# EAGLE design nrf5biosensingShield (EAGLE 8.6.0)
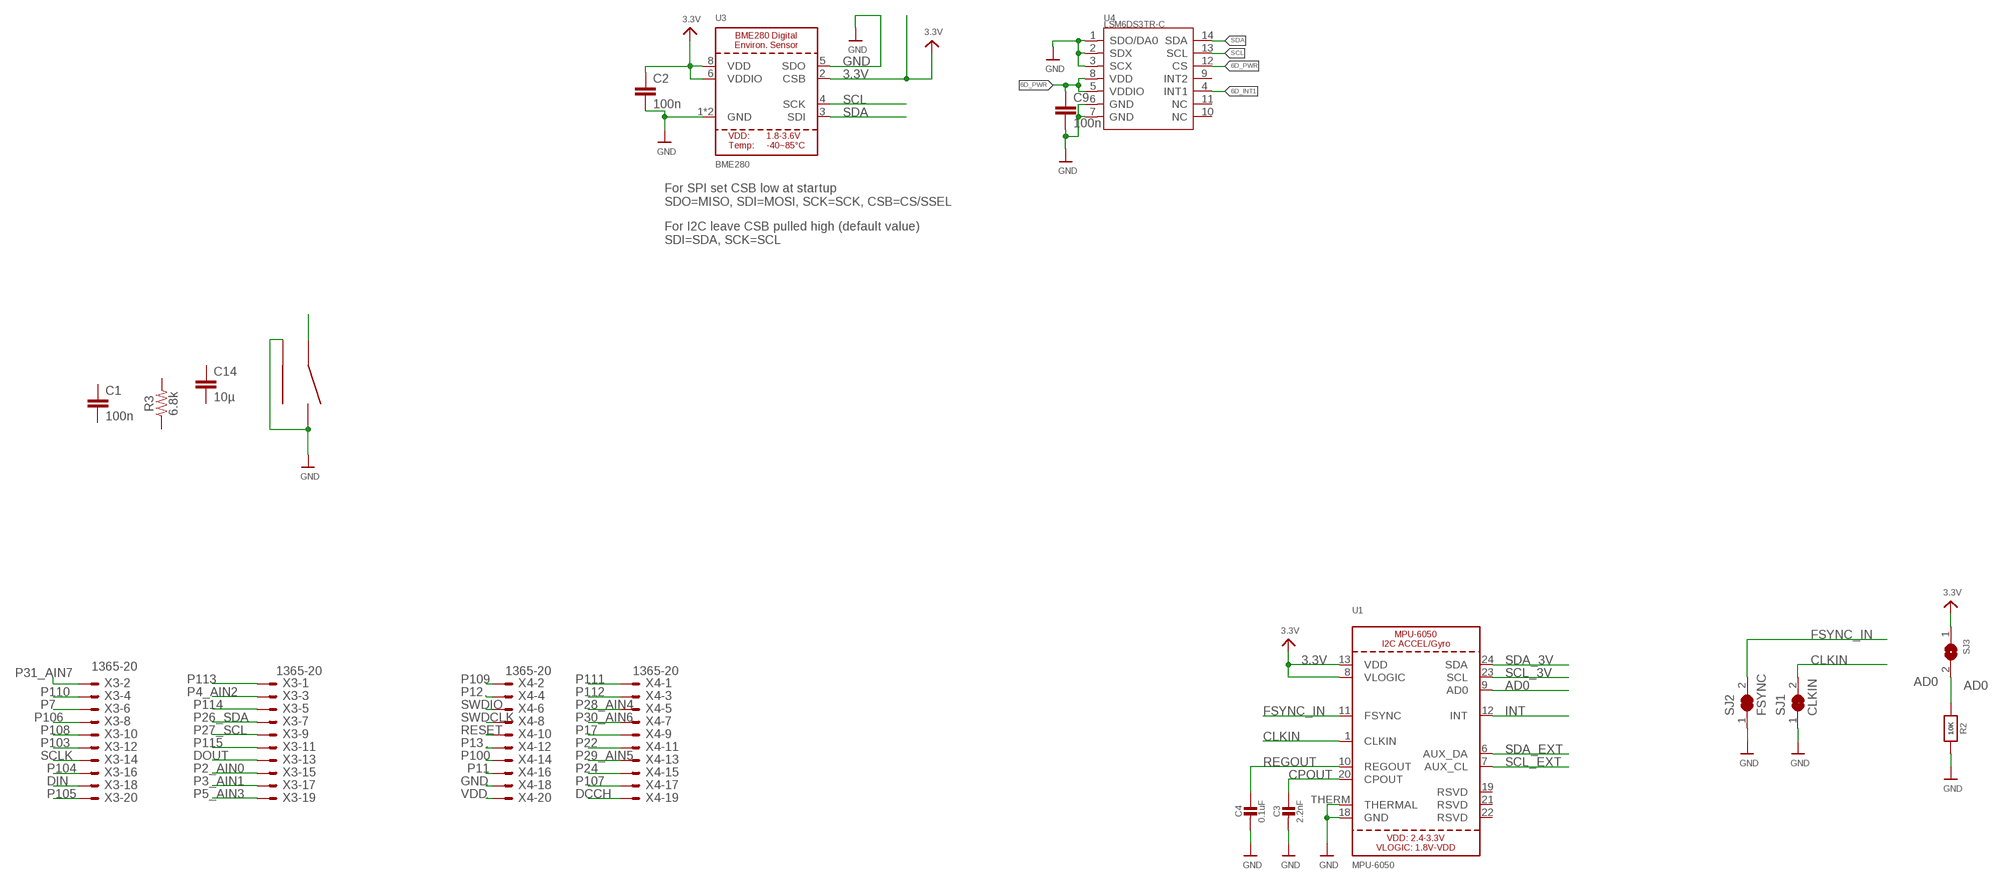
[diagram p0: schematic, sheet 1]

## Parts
C1  100n  CAP-0402-TIGHT  [0402-TIGHT]
C2  100n  C-EUC0402  [C0402]
C3  2.2nF  CAP_CERAMIC0603_NO  [0603-NO]
C4  0.1uF  CAP_CERAMIC0603_NO  [0603-NO]
C9  100n  C-EUC0402  [C0402]
C14  10µ  C-EUC0603  [C0603]
R2  10K  RESISTOR_0603_NOOUT  [0603-NO]
R3  6.8k  RESISTOR0402T  [0402-TIGHT]
S1  LS12T2  [LS12T2]
SJ1  CLKIN  SOLDERJUMPER_CLOSED  [SOLDERJUMPER_CLOSEDWIRE]
SJ2  FSYNC  SOLDERJUMPER_CLOSED  [SOLDERJUMPER_CLOSEDWIRE]
SJ3  SOLDERJUMPER  [SOLDERJUMPER_ARROW_NOPASTE]
U1  MPU-6050  [QFN24_4MM_SMSC]
U3  BME280  [BME280]
U4  LSM6DS3TR-C  SENSOR-LSM6DS3TR-C  [LGA14-0.5-2.5X3X0.86MM]
X3  1365-20  [1365-20]
X4  1365-20  [1365-20]

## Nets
3.3V [power]: C2.1 SJ3.1 U1.8(VLOGIC) U1.13(VDD) U3.2(CSB) U3.6(VDDIO) U3.8(VDD)
6D_INT1: U4.4(INT1)
6D_PWR: C9.1 U4.5(VDDIO) U4.8(VDD) U4.12(CS)
AD0: R2.1 SJ3.2 U1.9(AD0)
BUT: S1.2
CLKIN: SJ1.2 U1.1(CLKIN)
CPOUT: C3.1 U1.20(CPOUT)
DCCH: X4.19
DIN: X3.18
DOUT: X3.13
FSYNC_IN: SJ2.2 U1.11(FSYNC)
GND: C2.2 C3.2 C4.2 C9.2 R2.2 S1.1 S1.FRAME(FRM) SJ1.1 SJ2.1 U1.18(GND) U1.THERM(THERMAL) U3.1(GND) U3.5(SDO) U3.7(GND) U4.1(SDO/DA0) U4.2(SDX) U4.3(SCX) U4.6(GND) U4.7(GND) X4.18
INT: U1.12(INT)
P2_AIN0: X3.15
P3_AIN1: X3.17
P4_AIN2: X3.3
P5_AIN3: X3.19
P7: X3.6
P11: X4.16
P12: X4.4
P13: X4.12
P17: X4.9
P22: X4.11
P24: X4.15
P26_SDA: X3.7
P27_SCL: X3.9
P28_AIN4: X4.5
P29_AIN5: X4.13
P30_AIN6: X4.7
P31_AIN7: X3.2
P100: X4.14
P103: X3.12
P104: X3.16
P105: X3.20
P106: X3.8
P107: X4.17
P108: X3.10
P109: X4.2
P110: X3.4
P111: X4.1
P112: X4.3
P113: X3.1
P114: X3.5
P115: X3.11
REGOUT: C4.1 U1.10(REGOUT)
RESET: X4.10
SCL: U3.4(SCK) U4.13(SCL)
SCL_3V: U1.23(SCL)
SCL_EXT: U1.7(AUX_CL)
SCLK: X3.14
SDA: U3.3(SDI) U4.14(SDA)
SDA_3V: U1.24(SDA)
SDA_EXT: U1.6(AUX_DA)
SWDCLK: X4.8
SWDIO: X4.6
VDD: X4.20
Unconnected: C1.1 C1.2 C14.1 C14.2 R3.1 R3.2 U1.19(RSVD) U1.21(RSVD) U1.22(RSVD) U4.9(INT2) U4.10(NC) U4.11(NC)

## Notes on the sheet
- For SPI set CSB low at startup
  SDO=MISO, SDI=MOSI, SCK=SCK, CSB=CS/SSEL
- For I2C leave CSB pulled high (default value)
  SDI=SDA, SCK=SCL

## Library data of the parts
C1 = SparkFun-Capacitors:CAP
C2 C9 C14 = rcl:C-EU: CAPACITOR, European symbol
C3 C4 = microbuilder:CAP_CERAMIC: Ceramic Capacitors
R2 = microbuilder:RESISTOR: Resistors
R3 = SparkFun-Resistors:RESISTOR: Generic Resistor Package
S1 = LS12T2:LS12T2
SJ1 SJ2 = microbuilder:SOLDERJUMPER_CLOSED: Solder Jumper - Closed
SJ3 = microbuilder:SOLDERJUMPER: SMD Solder JUMPER; BOM: EXCLUDE
U1 = microbuilder:MPU-6050: MPU-6050 3-Axis Accelerometer/Gyroscope
U3 = microbuilder:BME280: BME280 - Environmental Sensor (I2C + SPI)
U4 = Making:SENSOR-LSM6DS3TR-C
X3 X4 = con-leotronics:1365-20: DUAL ROW STRAIGHT HEADER 1364 SERIES. 1.27mm x 1.27mm. Without Fixing Post. SMT Source: http://www.leotronics.co.uk/Conexcon/Data%20Sheets/sec.%20A/1364ing.pdf; OC_FARNELL: unknown; OC_NEWARK: unknown

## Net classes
1 power: width 0.254 mm

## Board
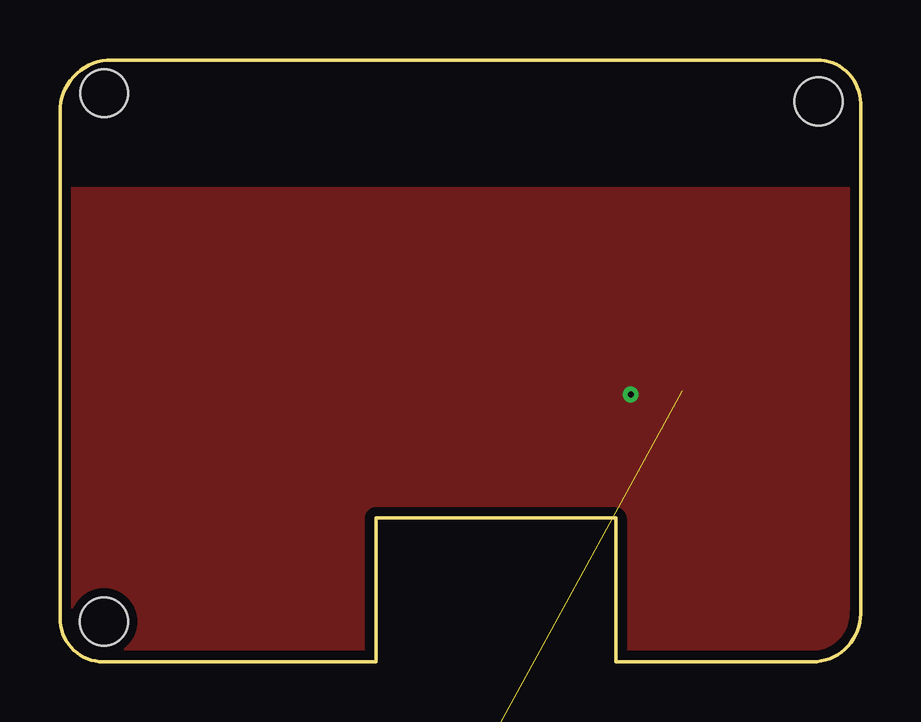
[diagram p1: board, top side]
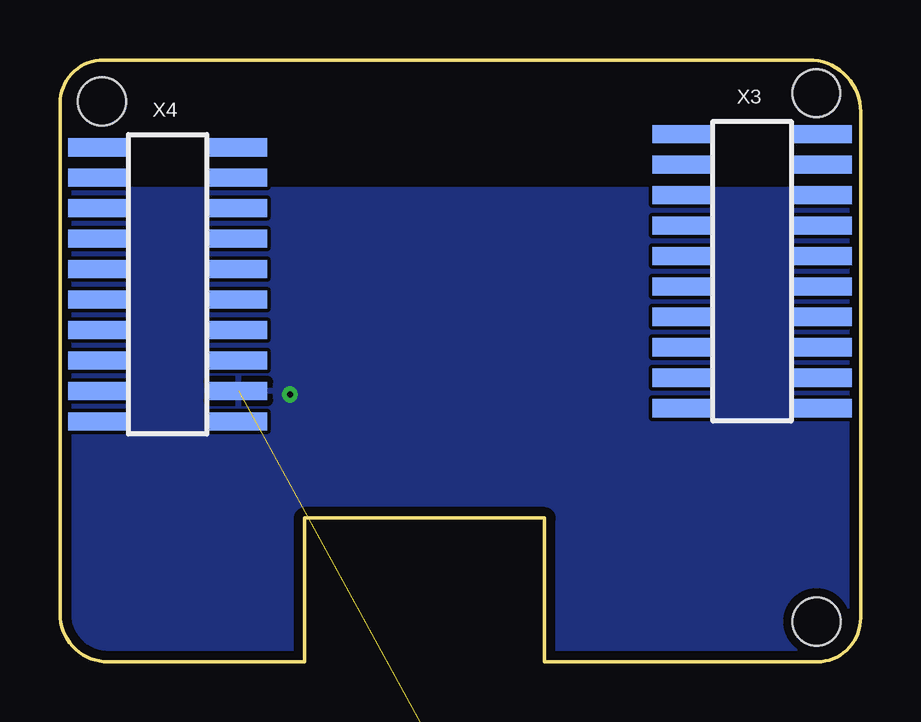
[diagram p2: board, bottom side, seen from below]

Size 33.38 x 25.1 mm. Coordinates in mm from the lower left corner, seen from the top.
Outline: 33.38,2.01 arc-90 31.37,0 23.18,0 23.18,6 13.18,6 13.18,0 1.8,0 arc-90 0,1.83 0,22.94 arc-90 2.16,25.1 31.55,25.1 arc-90 33.38,23.29 33.38,2.01
Copper layers (1*16): Top 0.035mm / dielectric 1.5mm / Bottom 0.035mm
Design rules "default *": minimum track width 6mil, minimum drill 0.35mm, track to track 6mil, track to pad 6mil, pad to pad 6mil, via to via 6mil, smd to smd 6mil, copper to edge 15mil, drill to drill 6mil, minimum pad ring 10mil, minimum via ring 8mil, stop-mask expansion 4mil, vias tented up to drill 20mil, thermal gap 10mil
Holes 2 mm at 1.84,23.71 31.62,23.36 1.83,1.67

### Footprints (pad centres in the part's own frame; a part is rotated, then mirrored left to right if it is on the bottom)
0402-TIGHT = smd 0.6 x 0.6: 1 -0.5,0; 2 0.5,0
C0402 = smd 0.7 x 0.9: 1 -0.65,0; 2 0.65,0
0603-NO = smd 1.075 x 1: 1 -0.85,0; 2 0.85,0
C0603 = smd 1.1 x 1: 1 -0.85,0; 2 0.85,0
LS12T2 = smd 1.1 x 0.7: 1 -1.45,1.4; 2 -1.45,-1.4 | smd 1.1 x 1.4: FRAME -1.6,0 | drill 0.6 pad 1.016 square: P$4 -0.1,-1.825; P$5 -0.1,1.825
SOLDERJUMPER_CLOSEDWIRE = smd 1.168 x 1.6: 1 -0.762,0; 2 0.762,0 | smd 0.635 x 0.203: WIRE 0,0
SOLDERJUMPER_ARROW_NOPASTE = smd 0.762 x 1.524: 1 -1.016,0; 2 1.016,0
QFN24_4MM_SMSC = smd 0.8 x 0.28: 1 -2,1.25; 2 -2,0.75; 3 -2,0.25; 4 -2,-0.25; 5 -2,-0.75; 6 -2,-1.25; 13 2,-1.25; 14 2,-0.75; 15 2,-0.25; 16 2,0.25; 17 2,0.75; 18 2,1.25 | smd 0.28 x 0.8: 7 -1.25,-2; 8 -0.75,-2; 9 -0.25,-2; 10 0.25,-2; 11 0.75,-2; 12 1.25,-2; 19 1.25,2; 20 0.75,2; 21 0.25,2; 22 -0.25,2; 23 -0.75,2; 24 -1.25,2 | smd 2.5 x 2.5: THERM 0,0
BME280 = smd 0.7 x 0.35: 1 1.025,0.975; 2 1.025,0.325; 3 1.025,-0.325; 4 1.025,-0.975; 5 -1.025,-0.975; 6 -1.025,-0.325; 7 -1.025,0.325; 8 -1.025,0.975
LGA14-0.5-2.5X3X0.86MM = smd 0.6 x 0.25: 1 -1.2,0.75; 2 -1.2,0.25; 3 -1.2,-0.25; 4 -1.2,-0.75; 8 1.2,-0.75; 9 1.2,-0.25; 10 1.2,0.25; 11 1.2,0.75 | smd 0.25 x 0.6: 5 -0.5,-0.95; 6 0,-0.95; 7 0.5,-0.95; 12 0.5,0.95; 13 0,0.95; 14 -0.5,0.95
1365-20 = smd 0.76 x 2.4: 1 -5.715,-2.95; 2 -5.715,2.95; 3 -4.445,-2.95; 4 -4.445,2.95; 5 -3.175,-2.95; 6 -3.175,2.95; 7 -1.905,-2.95; 8 -1.905,2.95; 9 -0.635,-2.95; 10 -0.635,2.95; 11 0.635,-2.95; 12 0.635,2.95; 13 1.905,-2.95; 14 1.905,2.95; 15 3.175,-2.95; 16 3.175,2.95; 17 4.445,-2.95; 18 4.445,2.95; 19 5.715,-2.95; 20 5.715,2.95

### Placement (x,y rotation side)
C1  not placed on the board
C2  not placed on the board
C3  not placed on the board
C4  not placed on the board
C9  not placed on the board
C14  not placed on the board
R2  not placed on the board
R3  not placed on the board
S1  not placed on the board
SJ1  not placed on the board
SJ2  not placed on the board
SJ3  not placed on the board
U1  not placed on the board
U3  not placed on the board
U4  not placed on the board
X3  4.53,16.29 270 bottom
X4  28.89,15.74 270 bottom

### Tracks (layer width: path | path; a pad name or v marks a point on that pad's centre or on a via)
3.3V  (6 unrouted)
6D_PWR  (3 unrouted)
AD0  (2 unrouted)
CLKIN  (1 unrouted)
CPOUT  (1 unrouted)
FSYNC_IN  (1 unrouted)
GND  (via drill 0.25)  (19 unrouted)
  other vias: 23.79,11.15
  pour Top: 33.95,19.72 -1.61,19.72 -1.61,8.29 -1.61,-0.6 33.95,-0.6
  pour Bottom: -3.2,19.72 34.9,19.72 34.9,-1.55 -3.2,-1.55
REGOUT  (1 unrouted)
SCL  (1 unrouted)
SDA  (1 unrouted)

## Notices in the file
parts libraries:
SparkFun-Capacitors: Licensing: Creative Commons ShareAlike 4.0 International - https://creativecommons.org/licenses/by-sa/4.0
microbuilder: This work is placed in the public domain, and may be freely used for commercial and non-commercial work with the following conditions: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
